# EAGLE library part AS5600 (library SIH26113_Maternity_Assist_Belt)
ams-OSRAM AS5600-ASOM 12-bit contactless magnetic rotary position sensor, SOIC-8. Fixed I2C address 0x36. Pin map from AS5600 DS000365 v1-06 Figure 4.
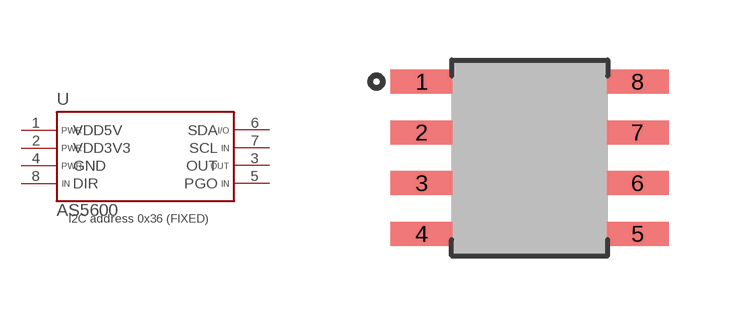
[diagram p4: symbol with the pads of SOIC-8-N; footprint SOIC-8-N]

Designator prefix U

## AS5600  [SOIC-8-N]
1  VDD5V  pwr
2  VDD3V3  pwr
3  OUT  out
4  GND  pwr
5  PGO  in
6  SDA
7  SCL  in
8  DIR  in

## Footprint SOIC-8-N (pad centres in mm)
SOIC-8 narrow (150 mil body). Body 4.90 x 3.90 mm, lead span 6.00 mm, 1.27 mm pitch. Lands 1.55 x 0.60 mm at 5.40 mm span (IPC-7351B SOIC127P600X175-8N Nominal).
smd 1.55 x 0.6: 1 -2.7,1.905; 2 -2.7,0.635; 3 -2.7,-0.635; 4 -2.7,-1.905; 5 2.7,-1.905; 6 2.7,-0.635; 7 2.7,0.635; 8 2.7,1.905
